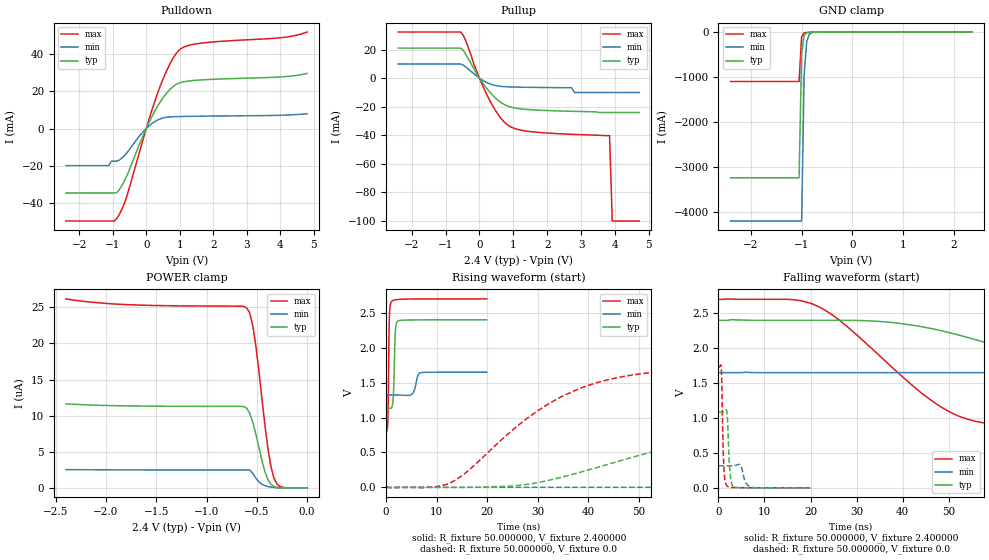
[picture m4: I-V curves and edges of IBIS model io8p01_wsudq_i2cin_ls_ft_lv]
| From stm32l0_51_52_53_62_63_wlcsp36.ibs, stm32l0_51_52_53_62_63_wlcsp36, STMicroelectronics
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|   Model io8p01_wsudq_i2cin_ls_ft_lv
[Model]  io8p01_wsudq_i2cin_ls_ft_lv
Model_type I/O
Polarity   Non-Inverting
Enable   Active-Low
Vinl =   0.720000V
Vinh =   1.680000V
Vmeas =  1.200000V
Cref =   50.000000pF
Rref =   100.000000M
Vref =   0.0V
C_comp   2.943600pF   2.919700pF   2.965100pF
[Temperature Range]   25.000000   0.105000k   -40.000000
[Pullup Reference]   2.400000V   1.650000V   2.700000V
[Pulldown Reference]   0.0V   0.0V   0.0V
[POWER Clamp Reference]   2.400000V   1.650000V   2.700000V
[GND Clamp Reference]   0.0V   0.0V   0.0V
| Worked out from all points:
|   slope of the pulldown table from 0 to 0.36 V, typ, clamps not added: 28.5 ohm
|   slope of the pullup table from 0 to 0.36 V, typ, clamps not added: 32.2 ohm
|   GND clamp passes 1 mA (typ) near -0.65 V on its own axis
|   rising waveform, R_fixture 50.000000, V_fixture 2.400000: 20-80 % time 286ps typ, 639ps min, 195ps max; typ from 1.14 V to 2.4 V
|   rising waveform, R_fixture 50.000000, V_fixture 0.0: 20-80 % time 39.7ns typ, 106ns min, 19.4ns max; typ from 0 V to 1.08 V
|   falling waveform, R_fixture 50.000000, V_fixture 2.400000: 20-80 % time 40.7ns typ, 106ns min, 20.1ns max; typ from 2.4 V to 1.14 V
|   falling waveform, R_fixture 50.000000, V_fixture 0.0: 20-80 % time 483ps typ, 854ps min, 380ps max; typ from 1.08 V to 0 V
[Pulldown]
|Voltage   I(typ)   I(min)   I(max)
-2.4V     -34.71mA   -20mA      -49.82mA
-1.12V    -34.71mA   -20mA      -49.82mA
-1.04V    -34.71mA   -17.6mA    -49.82mA
-880mV    -34.55mA   -17.6mA    -48.46mA
-560mV    -24.65mA   -12.68mA   -35.33mA
0V        225fA      0A         140fA
400mV     13.84mA    5.066mA    22.03mA
720mV     21.25mA    6.254mA    35.26mA
1.04V     24.82mA    6.464mA    43.03mA
1.6V      26.11mA    6.627mA    45.88mA
4V        27.76mA    7.125mA    48.87mA
4.8V      29.64mA    7.94mA     51.96mA
[Pullup]
|Voltage   I(typ)   I(min)   I(max)
-2.4V     21.07mA    9.995mA    32.35mA
-560mV    21.07mA    9.995mA    32.35mA
-400mV    16.53mA    7.728mA    25.89mA
-80mV     3.011mA    1.496mA    4.671mA
320mV     -10.16mA   -4.078mA   -16.34mA
640mV     -17.08mA   -5.718mA   -28.28mA
960mV     -20.45mA   -6.129mA   -34.49mA
1.76V     -22.39mA   -6.471mA   -37.97mA
2.8V      -23.2mA    -10mA      -39.35mA
3.84V     -24mA      -10mA      -40.2mA
3.92V     -24mA      -10mA      -100mA
4.72V     -24mA      -10mA      -100mA
[GND_clamp]
|Voltage   I(typ)   I(min)   I(max)
-2.4V     -3.237A    -4.198A    -1.1A
-1.05V    -3.237A    -4.198A    -1.1A
-1V       -475.8mA   -4.198A    -104.2mA
-950mV    -76.24mA   -935.4mA   -18.39mA
-900mV    -16.61mA   -212.9mA   -9.105mA
-850mV    -6.547mA   -50.94mA   -6.589mA
-800mV    -3.998mA   -13.81mA   -4.86mA
-650mV    -1.043mA   -1.182mA   -1.146mA
2.35V     0A         0A         0A
[POWER_clamp]
|Voltage   I(typ)   I(min)   I(max)
-2.4V     11.64uA    2.525uA    26.17uA
-1.86V    11.37uA    2.488uA    25.42uA
-600mV    11.04uA    2.474uA    24.9uA
-570mV    10.3uA     2.473uA    24.21uA
-540mV    9.097uA    2uA        22.48uA
-510mV    7.497uA    1.35uA     19.73uA
-450mV    3.845uA    512.5nA    12.52uA
-390mV    1.154uA    175.5nA    5.528uA
-360mV    508.2nA    102.8nA    2.997uA
-330mV    204.4nA    60.39nA    1.375uA
-270mV    0A         0A         194.9nA
0V        0A         0A         0A
[Ramp]
| variable   typ   min   max
dV/dt_r  0.65076/39.66223n   0.18980/0.10642u   1.03800/19.37179n
dV/dt_f  0.75690/40.67914n   0.19476/0.10534u   1.13815/20.05098n
R_load = 50.000000
[Rising Waveform]
R_fixture= 50.000000
V_fixture= 2.400000
V_fixture_min= 1.650000
V_fixture_max= 2.700000
|time   V(typ)   V(min)   V(max)
0s        1.139V     1.322V     800.5mV
360.4ps   1.137V     1.322V     1.013V
640.6ps   1.134V     1.322V     2.435V
1.081ns   1.143V     1.322V     2.662V
1.441ns   1.335V     1.322V     2.68V
1.842ns   2.258V     1.322V     2.686V
2.242ns   2.377V     1.322V     2.69V
5.165ns   2.398V     1.339V     2.698V
6.887ns   2.399V     1.642V     2.699V
19.94ns   2.4V       1.65V      2.7V
[Rising Waveform]
R_fixture= 50.000000
V_fixture= 0.0
V_fixture_min= 0.0
V_fixture_max= 0.0
|time   V(typ)   V(min)   V(max)
0s        8.881uV    -3.863uV   -11.56uV
13.01ns   -216.8uV   -47.52uV   76.05mV
28.03ns   43.79mV    -46.16uV   994.5mV
38.04ns   208.2mV    -45.87uV   1.407V
48.05ns   415.6mV    -42.37uV   1.601V
61.06ns   656.3mV    29.07uV    1.691V
85.09ns   924.7mV    1.083mV    1.726V
124.1ns   1.059V     43.48mV    1.73V
254.3ns   1.085V     267.4mV    1.73V
498.5ns   1.085V     316.6mV    1.73V
[Falling Waveform]
R_fixture= 50.000000
V_fixture= 2.400000
V_fixture_min= 1.650000
V_fixture_max= 2.700000
|time   V(typ)   V(min)   V(max)
0s        2.4V       1.65V      2.7V
20.02ns   2.4V       1.65V      2.644V
26.03ns   2.4V       1.65V      2.413V
49.05ns   2.24V      1.65V      1.131V
56.06ns   2.119V     1.65V      951mV
68.07ns   1.871V     1.65V      861.4mV
95.1ns    1.392V     1.65V      814.3mV
135.1ns   1.201V     1.635V     802.5mV
286.3ns   1.139V     1.381V     800.5mV
498.5ns   1.139V     1.322V     800.5mV
[Falling Waveform]
R_fixture= 50.000000
V_fixture= 0.0
V_fixture_min= 0.0
V_fixture_max= 0.0
|time   V(typ)   V(min)   V(max)
0s        1.085V     316.6mV    1.73V
600.6ps   1.085V     316.6mV    1.72V
1.121ns   1.084V     316.6mV    366mV
1.361ns   1.091V     316.6mV    125.9mV
1.762ns   1.111V     316.6mV    33.22mV
2.482ns   242.5mV    316.4mV    8.286mV
3.243ns   17.74mV    316.7mV    4.405mV
4.805ns   2.321mV    322.6mV    2.04mV
7.207ns   940.3uV    8.295mV    746.8uV
19.94ns   8.881uV    -3.863uV   -11.56uV
